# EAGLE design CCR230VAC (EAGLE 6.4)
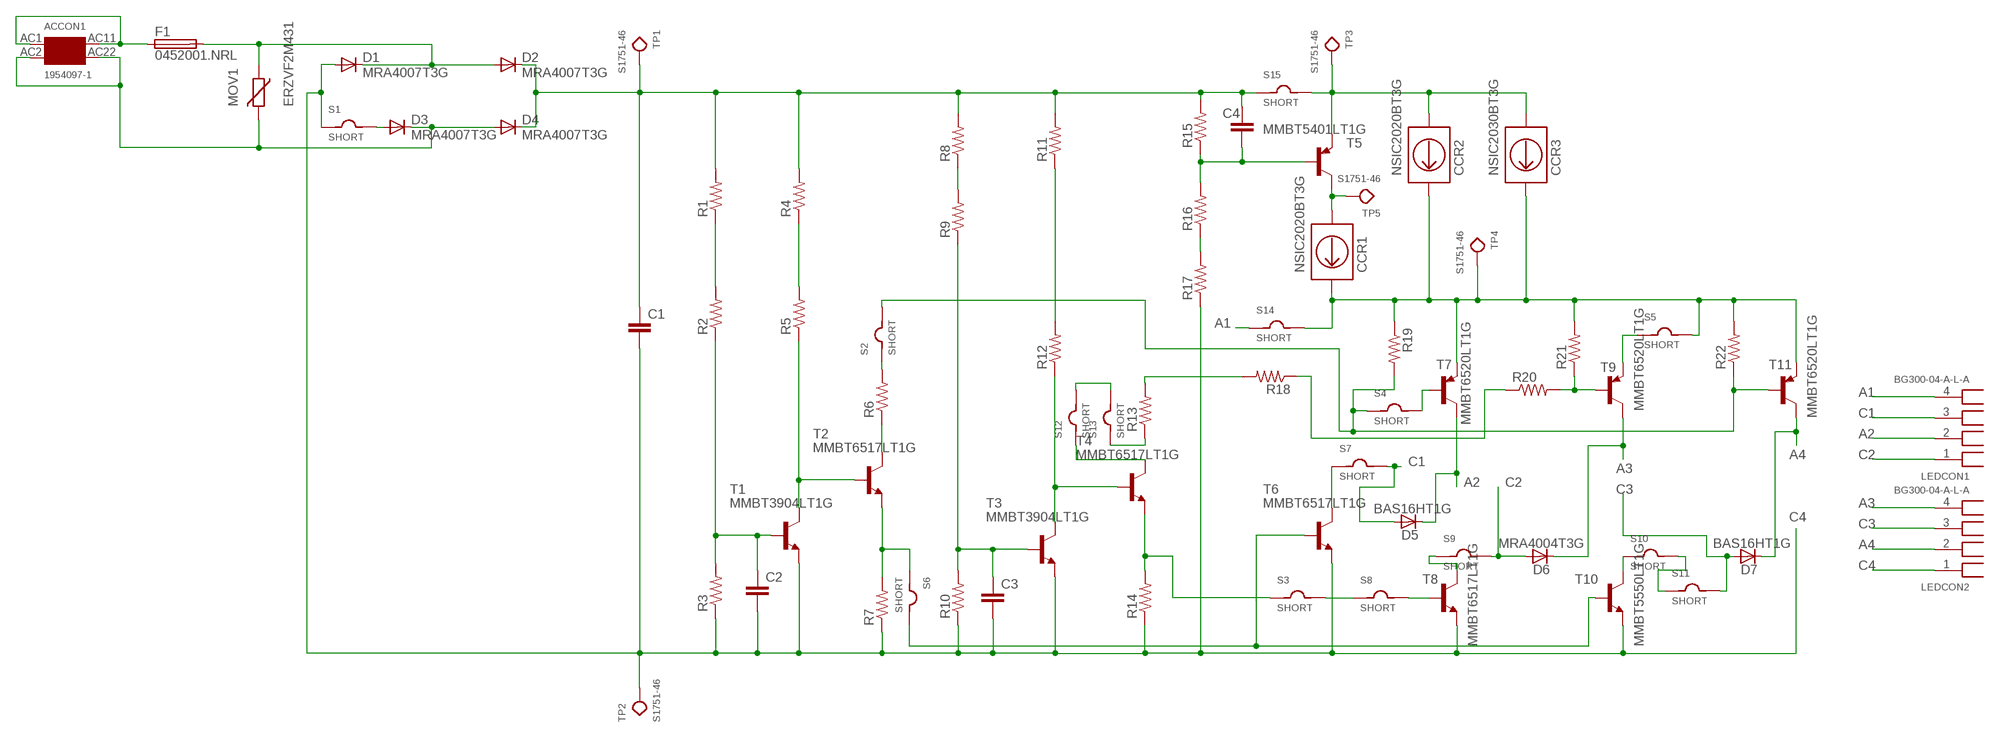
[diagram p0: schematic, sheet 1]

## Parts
ACCON1  1954097-1  [LEDCON_SMT]
C1  C-EUC1206K  [C1206K]
C2  C-EUC0805K  [C0805K]
C3  C-EUC0805K  [C0805K]
C4  C-EUC0805K  [C0805K]
CCR1  NSIC2020BT3G  NSIC2030BT3G  [SMB]
CCR2  NSIC2020BT3G  NSIC2030BT3G  [SMB]
CCR3  NSIC2030BT3G  [SMB]
D1  MRA4007T3G  MRA4004T3G  [SMA]
D2  MRA4007T3G  MRA4004T3G  [SMA]
D3  MRA4007T3G  MRA4004T3G  [SMA]
D4  MRA4007T3G  MRA4004T3G  [SMA]
D5  BAS16HT1G  [SOD323-R]
D6  MRA4004T3G  [SMA]
D7  BAS16HT1G  [SOD323-R]
F1  0452001.NRL  [SMTFUSE]
LEDCON1  BG300-04-A-L-A  [LEDCON_4_F]
LEDCON2  BG300-04-A-L-A  [LEDCON_4_F]
MOV1  ERZVF2M431  ERZVF2M241  [CU3225K]
R1  R-US_R1206  [R1206]
R2  R-US_R1206  [R1206]
R3  R-US_R1206  [R1206]
R4  R-US_R1206  [R1206]
R5  R-US_R1206  [R1206]
R6  R-US_R1206  [R1206]
R7  R-US_R1206  [R1206]
R8  R-US_R1206  [R1206]
R9  R-US_R1206  [R1206]
R10  R-US_R1206  [R1206]
R11  R-US_R1206  [R1206]
R12  R-US_R1206  [R1206]
R13  R-US_R1206  [R1206]
R14  R-US_R1206  [R1206]
R15  R-US_R1206  [R1206]
R16  R-US_R1206  [R1206]
R17  R-US_R1206  [R1206]
R18  R-US_R1206  [R1206]
R19  R-US_R1206  [R1206]
R20  R-US_R1206  [R1206]
R21  R-US_R1206  [R1206]
R22  R-US_R1206  [R1206]
S1  SHORT  [R2010]
S2  SHORT  [R2010]
S3  SHORT  [R2010]
S4  SHORT  [R2010]
S5  SHORT  [R2010]
S6  SHORT  [R2010]
S7  SHORT  [R2010]
S8  SHORT  [R2010]
S9  SHORT  [R2010]
S10  SHORT  [R2010]
S11  SHORT  [R2010]
S12  SHORT  [R2010]
S13  SHORT  [R2010]
S14  SHORT  [R2010]
S15  SHORT  [R2010]
T1  MMBT3904LT1G  [SOT23]
T2  MMBT6517LT1G  [SOT23]
T3  MMBT3904LT1G  [SOT23]
T4  MMBT6517LT1G  [SOT23]
T5  MMBT5401LT1G  [SOT23]
T6  MMBT6517LT1G  [SOT23]
T7  MMBT6520LT1G  [SOT23]
T8  MMBT6517LT1G  [SOT23]
T9  MMBT6520LT1G  [SOT23]
T10  MMBT5550LT1G  [SOT23]
T11  MMBT6520LT1G  [SOT23]
TP1  S1751-46  [TEST_SMT]
TP2  S1751-46  [TEST_SMT]
TP3  S1751-46  [TEST_SMT]
TP4  S1751-46  [TEST_SMT]
TP5  S1751-46  [TEST_SMT]

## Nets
A1: LEDCON1.4 S14.1
A2: D5.C LEDCON1.2 T7.3(C)
A3: D6.C LEDCON2.4 T9.3(C)
A4: D7.C LEDCON2.2 T11.3(C)
C1: D5.A LEDCON1.3 S7.2
C2: D6.A LEDCON1.1 S9.2
C3: D7.A LEDCON2.3 S11.2
C4: C1.2 C2.2 C3.2 D1.A LEDCON2.1 R3.1 R7.1 R10.1 R14.1 R17.1 S1.1 T1.2(E) T3.2(E) T6.2(E) T8.2(E) T10.2(E) TP2.P$1
CONECT: R19.2 R22.1 S2.2 S4.1 T11.1(B)
DDD: CCR1.C CCR2.C CCR3.C R19.1 R21.2 R22.2 S5.2 S14.2 T7.2(E) T11.2(E) TP4.P$1
N$1: ACCON1.AC1 ACCON1.AC11 F1.P$1
N$2: ACCON1.AC2 ACCON1.AC22 D3.C D4.A MOV1.2
N$3: D1.C D2.A F1.P$2 MOV1.1
N$4: D3.A S1.2
N$5: C4.2 R15.1 R16.2 T5.1(B)
N$6: R1.1 R2.2
N$7: C1.1 C4.1 D2.C D4.C R1.2 R4.2 R8.2 R11.2 R15.2 S15.1 TP1.P$1
N$8: R4.1 R5.2
N$9: C2.1 R2.1 R3.2 T1.1(B)
N$10: R5.1 T1.3(C) T2.1(B)
N$11: R16.1 R17.2
N$12: S6.2 T6.1(B) T10.1(B)
N$13: R6.2 S2.1
N$14: R6.1 T2.3(C)
N$15: R8.1 R9.2
N$16: C3.1 R9.1 R10.2 T3.1(B)
N$17: R20.2 R21.1 T9.1(B)
N$18: CCR1.A T5.3(C) TP5.P$1
N$19: R11.1 R12.2
N$20: R12.1 T3.3(C) T4.1(B)
N$21: R14.2 S3.1 T4.2(E)
N$22: S12.1 T4.3(C)
N$23: S3.2 S8.1
N$24: S5.1 T9.2(E)
N$25: R13.2 R18.2
N$26: R18.1 R20.1
N$27: S4.2 T7.1(B)
N$28: R7.2 S6.1 T2.2(E)
N$29: S7.1 T6.3(C)
N$30: S8.2 T8.1(B)
N$31: S9.1 T8.3(C)
N$32: S10.1 T10.3(C)
N$33: S10.2 S11.1
N$34: R13.1 S13.1
N$35: S12.2 S13.2
N$36: CCR2.A CCR3.A S15.2 T5.2(E) TP3.P$1

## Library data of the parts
ACCON1 = CCR_120VAC_LIB:1954097-1
C1-C4 = resistor:C-EU: CAPACITOR, European symbol
CCR1-CCR3 = CCR_120VAC_LIB:NSIC2030BT3G
D1-D4 D6 = CCR_120VAC_LIB:MRA4004T3G
D5 D7 = CCR_120VAC_LIB:BAS16HT1G
F1 = CCR_120VAC_LIB:0452001.NRL
LEDCON1 LEDCON2 = CCR_120VAC_LIB:BG300-04-A-L-A
MOV1 = CCR_120VAC_LIB:ERZVF2M241
R1-R22 = resistor:R-US_: RESISTOR, American symbol
S1-S15 = CCR_120VAC_LIB:SHORT
T1 T3 = CCR_120VAC_LIB:MMBT3904LT1G
T2 T4 T6 T8 = CCR_120VAC_LIB:MMBT6517LT1G
T5 = CCR_120VAC_LIB:MMBT5401LT1G
T7 T9 T11 = CCR_120VAC_LIB:MMBT6520LT1G
T10 = CCR_120VAC_LIB:MMBT5550LT1G
TP1-TP5 = CCR_120VAC_LIB:S1751-46

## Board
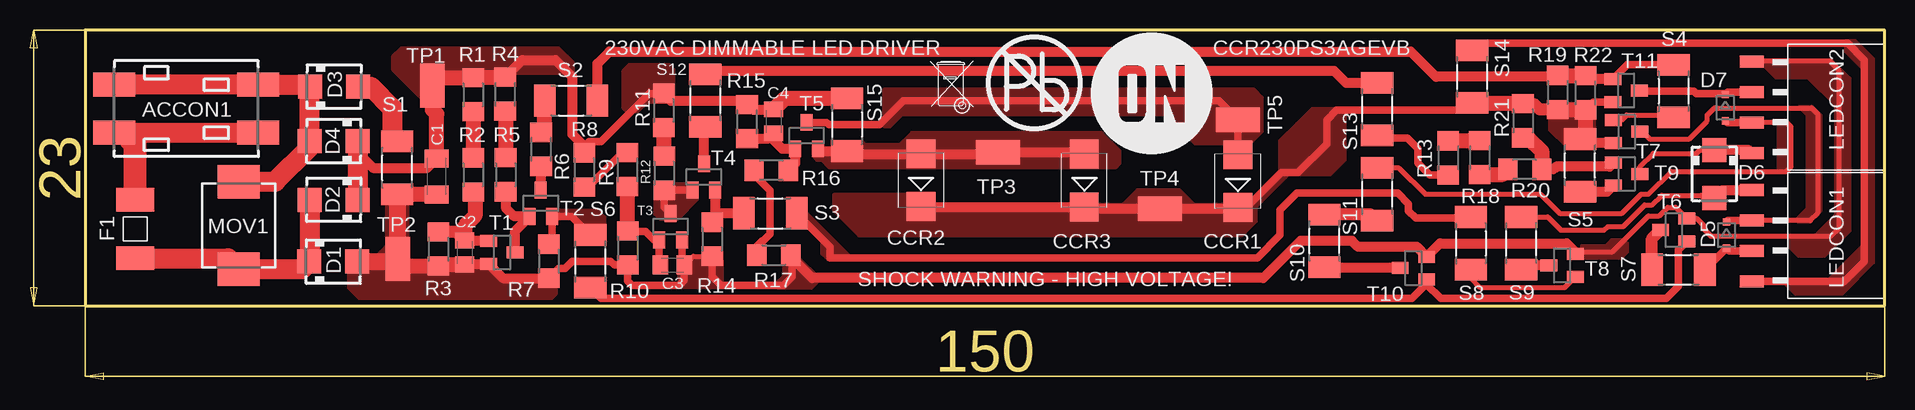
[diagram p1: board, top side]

Size 154.6 x 29.2 mm. Coordinates in mm from the lower left corner, seen from the top.
Outline: 4.6,6.2 154.6,6.2 154.6,29.2 4.6,29.2 4.6,6.2
Copper layers (1*16): Top 0.035mm / dielectric 1.5mm / Bottom 0.035mm
Design rules "default": minimum track width 10mil, minimum drill 24mil, track to track 8mil, track to pad 8mil, pad to pad 8mil, via to via 8mil, smd to smd 8mil, copper to edge 1mil, drill to drill 8mil, minimum pad ring 10mil, minimum via ring 8mil, stop-mask expansion 4mil, vias tented up to drill 0mil, thermal gap 10mil

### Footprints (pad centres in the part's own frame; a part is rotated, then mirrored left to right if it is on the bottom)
LEDCON_SMT = smd 3.5 x 2: AC1 -6,2; AC2 -6,-2; AC11 6,2; AC22 6,-2
C1206K = smd 1.5 x 2: 1 -1.5,0; 2 1.5,0
C0805K = smd 1.3 x 1.6: 1 -1,0; 2 1,0
SMB = smd 2.4 x 2.4: A 2.2,0; C -2.2,0
SMA = smd 2 x 2: A 2,0; C -2,0
SOD323-R = smd 0.6 x 0.6: A 1.1,0; C -1.1,0
SMTFUSE = smd 1.96 x 3.15: P$1 -2.45,0; P$2 2.45,0
LEDCON_4_F = smd 2 x 1: 1 0,2.54; 2 0,0; 3 0,-2.54; 4 0,-5.08
CU3225K = smd 2.8 x 3.5: 1 -3.65,0; 2 3.65,0
R1206 = smd 1.6 x 1.803: 1 -1.422,0; 2 1.422,0
R2010 = smd 1.8 x 2.7: 1 -2.2,0; 2 2.2,0
SOT23 = smd 1 x 1.4: 1 -0.95,-1.1; 2 0.95,-1.1; 3 0,1.1
TEST_SMT = smd 3.65 x 2.05: P$1 0,0

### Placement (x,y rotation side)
ACCON1  13.03,22.62 180 top
C1  33.91,16.99 270 top
C2  36.24,10.64 270 top
C3  53.55,9.59 0 top
C4  61.99,21.56 270 top
CCR1  100.68,16.58 90 top
CCR2  74.28,16.66 90 top
CCR3  87.88,16.64 90 top
D1  25.29,9.87 0 top
D2  25.33,15.03 180 top
D3  25.35,24.47 0 top
D4  25.32,19.93 180 top
D5  141.41,12.09 270 top
D6  140.4,17.2 270 top
D7  141.31,22.71 270 top
F1  8.77,12.59 270 top
LEDCON1  143.5,13.3 0 top
LEDCON2  143.5,24 0 top
MOV1  17.39,12.9 90 top
R1  36.95,23.81 90 top
R2  36.95,17.11 90 top
R3  34.05,10.93 90 top
R4  39.6,23.85 90 top
R5  39.65,17.12 90 top
R6  42.6,19.24 90 top
R7  43.25,9.91 90 top
R8  46.2,17.53 90 top
R9  49.8,17.55 90 top
R10  49.82,11.01 90 top
R11  52.82,22.48 90 top
R12  52.87,17.25 90 top
R13  118.22,18.52 90 top
R14  56.87,11.74 90 top
R15  59.77,21.56 90 top
R16  61.78,17.48 0 top
R17  62,10.42 180 top
R18  120.84,18.56 90 top
R19  127.34,23.98 90 top
R20  124.6,17.56 0 top
R21  124.44,21.62 90 top
R22  129.66,23.96 270 top
S1  30.6,17.7 90 top
S2  45.1,23.3 0 top
S3  61.7,13.9 0 top
S4  137,24.1 270 top
S5  129.2,17.9 90 top
S6  46.7,9.9 270 top
S7  137.4,9.2 0 top
S8  120.1,11.4 270 top
S9  124.3,11.4 90 top
S10  107.9,11.6 90 top
S11  112.3,15.5 90 top
S12  56.3,23.3 90 top
S13  112.3,22.6 90 top
S14  120.2,25.3 270 top
S15  68.1,21.3 270 top
T1  39.34,10.64 270 top
T2  42.58,14.74 0 top
T3  53.4,12.79 0 top
T4  56.17,16.94 0 top
T5  64.74,20.39 0 top
T6  137.01,12.51 90 top
T7  133.09,20.72 270 top
T8  127.71,9.55 90 top
T9  133.09,17.19 270 top
T10  115.31,9.33 90 top
T11  133.04,24.15 270 top
TP1  33.55,24.55 270 top
TP2  30.65,10.1 270 top
TP3  80.7,19 0 top
TP4  94.2,14.3 0 top
TP5  100.7,21.7 0 top
U$1  [ON2]  93.5,23.9 0 top
U$2  [BIN2]  76.8,24.5 0 top
U$3  [PB1]  83.7,24.8 0 top

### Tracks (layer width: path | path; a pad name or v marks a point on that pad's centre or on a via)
A1
  Top 0.61: S14.1 120.8,28.1 151.5,28.1 152.9,26.7 152.9,9.9 151.22,8.22 LEDCON1.4
  pour Top: 146.2,8.2 146.2,8.1 147.1,7.2 151.1,7.2 153.7,9.8 153.7,26.8 152.3,28.2 152.2,28.3 151.3,28.3 151.3,27.4 152.7,26 152.7,11.2 149.9,8.4 146.2,8.4
A2
  Top 0.406: LEDCON1.2 148.4,13.3 149,13.9 149,22.2 148.5,22.7 140.4,22.7 139.8,22.1 139.8,21.6 138.3,20.1 135,20.1 134.38,20.72 T7.3
  Top 0.61: LEDCON1.2 141.52,13.3 D5.C
  pour Top: 147.3,13.2 148.4,13.2 149.3,14.1 149.3,22.1 148.6,22.8 147.4,22.8 148.1,22.1 148.1,14.3 147.3,13.5
A3
  Top 0.406: T9.3 134.19,17.79 135.3,18.9 138.9,18.9 139.2,19.2 D6.C
  Top 0.813: LEDCON2.4 143.22,19.2 D6.C
A4
  Top 0.61: LEDCON2.2 141.5,24 D7.C 141.22,23.9 138.9,23.9 138.7,24.1 134.19,24.1 T11.3
C1
  Top 0.61: S7.2 139.62,9.2 D5.A 141.64,10.76 LEDCON1.3
C2
  Top 0.406: S9.2 126.5,13.6 127.6,12.5 131.2,12.5 131.5,12.8 132.8,12.8 134.6,14.6 135.2,14.6 136,15.4 139.3,15.4 139.5,15.2 D6.A
  Top 0.813: D6.A 141.04,15.84 LEDCON1.1
C3
  Top 0.406: S11.2 114.1,17.7 116.3,15.5 125.9,15.5 127.5,13.9 132.7,13.9 134.3,15.5 134.9,15.5 136.8,17.4 146.4,17.4 146.8,17.8 146.8,21.1 146.44,21.46 LEDCON2.3
  Top 0.61: D7.A 141.46,21.46 LEDCON2.3
  pour Top: 145.7,21.4 145.7,17.4 146.4,17.4 146.8,17.8 146.8,21.1 146.4,21.5 145.8,21.5
C4
  Top 0.406: C3.2 55.28,10.32 R14.1 | 128.81,10.69 131.89,10.69 134.9,13.7 135.8,13.7 136.5,14.4 137.17,14.4 T6.2 138.94,13.46 139.5,12.9 139.5,12.6 140.1,12 150.1,12 150.8,12.7 150.8,25.8 150,26.6 143.56,26.6 LEDCON2.1
  Top 0.61: R7.1 44.06,9.3 44.6,9.3 45.2,9.9 48.4,9.9 48.71,9.59 R10.1 49.82,8.28 50.2,7.9 54.1,7.9 54.5,8.3 54.5,9.54 C3.2 54.35,9.79 T3.2 | R14.1 56.87,8.63 57.6,7.9 62.8,7.9 63.5,8.6 63.5,10.34 R17.1
  Top 0.813: C2.2 38.19,9.64 T1.2 39.44,8.49 R7.1 | T8.2 128.81,10.69 128.1,11.4 117.53,11.4 T10.2 115.59,11.1 110.7,11.1 110.2,11.6 105.9,11.6 102.8,8.5 65.2,8.5 63.42,10.28 R17.1
  Top 1.27: S1.1 C1.2 | TP2.P$1 31.24,9.51 R3.1 34.18,9.64 C2.2
  Top 1.422: S1.1 30.6,10.15 TP2.P$1 30.42,9.87 D1.A
  pour Top (no thermals): 26.5,10 26.5,7.7 27.4,6.8 43.5,6.8 43.9,7.2 43.9,8.3 43.5,8.7 39.3,8.7 38.2,9.8 31.8,9.8 31.5,10.1 31.5,15 31.3,15.2 29.9,15.2 29.7,15 29.7,11.2 28.9,10.4 26.9,10.4
  pour Top (no thermals): 54.1,10.2 57.5,10.2 57.7,10 57.7,7.9 57.5,7.7 54.3,7.7 54.1,7.9
  pour Top (no thermals): 129.3,10.2 132.7,10.2 133.2,10.7 133.2,11.4 132.9,11.7 131.8,11.7 131.3,11.2 129.3,11.2
  pour Top (no thermals): 144.3,26.7 150.2,26.7 151.7,25.2 151.7,12.4 149.6,10.3 147.4,10.3 146.7,11 146.7,11.7 147.1,12.1 148.8,12.1 150.5,13.8 150.5,22.9 148.2,25.2 145.5,25.2 144.5,26.2 144.3,26.2
  pour Top (no thermals): 62.8,9.8 62.8,8.7 62.2,8.1 62.2,7.8 62.3,7.7 65.2,7.7 65.8,8.3 65.8,8.5 64.1,10.2 64.1,11.2 62.8,11.2
CONECT
  Top 0.61: T11.1 133.14,26.3 S4.1
  Top 0.813: S2.2 47.3,26.4 48.3,27.4 115.1,27.4 117.2,25.3 127.24,25.3 R19.2 | T11.1 129.94,25.1 R22.1
  Top 1.27: R19.2 129.64,25.4 R22.1
DDD
  Top 0.61: T11.2 130.32,23.2 R22.2 | CCR1.C 101.38,14.38 104.3,17.3 105.7,17.3 108.1,19.7 108.1,21.7 108.9,22.5 119.6,22.5 S14.2
  Top 0.813: T7.2 129.53,19.77 S5.2 | CCR2.C 74.3,14.44 CCR3.C 88.02,14.3 TP4.P$1 100.6,14.3 CCR1.C
  Top 1.016: R19.1 125.84,22.56 125.4,23 124.48,23 R21.2
  Top 1.27: R19.1 129.64,22.56 R22.2 129.66,20.56 S5.2 | R21.2 120.26,23.04 S14.2
  pour Top (no thermals): 126.7,23.1 130.2,23.1 130.4,22.9 130.4,19.7 130.2,19.5 128,19.5 126.7,20.8
  pour Top (no thermals): 67,15.5 74.5,15.5 75.3,14.7 91.1,14.7 92.3,15.9 95.8,15.9 97,14.7 101.4,14.7 104.2,17.5 104.2,20 105.6,21.4 106.9,22.7 108.6,22.7 109,22.7 109.6,22.1 109.6,18.3 108.4,17.1 104.9,17.1 102.2,14.4 102.2,13.2 101,12 69.1,12 67,14.1
N$1
  Top 1.676: ACCON1.AC11 7.85,20.62 ACCON1.AC1
  Top 1.93: F1.P$1 8.77,19.7 7.85,20.62
N$2
  Top 1.676: ACCON1.AC22 ACCON1.AC2 23.2,24.62 D3.C 23.32,24.44 D4.A 23.3,19.91 23.3,19.4 20.45,16.55 MOV1.2
N$3
  Top 1.676: F1.P$2 16.5,10.14 MOV1.1 22.67,9.25 D1.C 23.33,9.91 D2.A
N$4
  Top 1.676: D3.A 28.43,24.47 30.2,22.7 30.2,20.3 S1.2
N$5
  Top 0.813: R15.1 61.57,20.14 C4.2 61.99,20.01 62.7,19.3 T5.1 63.79,18.07 R16.2
N$6
  Top 1.27: R1.1 R2.2
N$7
  Top 0.61: R11.2 51.6,23.9 47.6,19.9 46.6,19.9 46.2,19.5
  Top 0.813: D4.C 27.32,18.98 28.6,17.7 33.12,17.7 C1.1 | R4.2 41.03,26.7 43.8,26.7 45.2,25.3 45.2,20.5 46.2,19.5 R8.2 | R11.2 53.42,23.3 59.2,23.3 59.52,22.98 R15.2 60.19,22.56 C4.1
  Top 1.27: C1.1 33.9,22.2 33.55,22.55 TP1.P$1 34.23,25.23 R1.2 36.99,25.27 R4.2 | C4.1 62.93,23.5 S15.1
  Top 1.676: D4.C D2.C
  pour Top (no thermals): 53.7,23.8 53.7,25.9 53.3,26.3 49.9,26.3 49.4,25.8 49.4,22.7 49.7,22.4 50.7,22.4 51.4,23.1 51.5,23.2 53.1,23.2
  pour Top (no thermals): 45.3,25.6 45.3,26.5 44.1,27.7 30.9,27.7 30.2,27 30.2,25.9 33.2,22.9 33.9,22.9 34.4,23.4 34.4,24.6 34.6,24.8 39.5,24.8 40.3,25.6
N$8
  Top 1.27: R4.1 39.65,22.38 R5.2
N$9
  Top 0.813: T1.1 36.29,11.59 C2.1
  Top 1.016: C2.1 35.53,12.35 R3.2
  Top 1.27: R2.1 37.1,15.54 37.1,13.7 36.24,12.84 C2.1
N$10
  Top 0.813: T1.3 40.44,12.45 T2.1 40.36,13.64 39.7,14.3 39.7,15.65 R5.1
N$11
  Top 0.61: R16.1 60.36,17.14 61.7,15.8 61.7,12.2 61.1,11.6 61,11.6 60.6,11.2 60.6,10.44 R17.2
N$12
  Top 0.61: T6.1 137.4,10.85 137.4,7.8 136.4,6.8 117.6,6.8 116.41,7.99 T10.1 116.41,8.01 115.2,6.8 47.6,6.8 S6.2
N$13
  Top 1.27: R6.2 42.9,20.96 S2.1
N$14
  Top 0.813: T2.3 42.6,15.86 R6.1
N$15
  Top 0.61: R8.1 46.51,16.11 49,18.6 49.43,18.6 R9.2
N$16
  Top 0.61: C3.1 52.45,9.69 T3.1 52.01,11.69 51.3,12.4 49.85,12.4 R10.2 | 49.82,16.11 R9.1
  Top 1.27: R10.2 49.82,16.11
N$17
  Top 0.813: T9.1 131.65,17.8 127.2,17.8 126.96,17.56 R20.2
  Top 1.27: R21.1 124.9,20.2 126,19.1 126,17.58 R20.2
N$18
  Top 0.61: T5.3 66.41,21.49 66.6,21.3 70.8,21.3 72.8,23.3 99.1,23.3 TP5.P$1 100.68,21.68 CCR1.A
  pour Top (no thermals): 71.2,24.3 102,24.3 102.7,23.6 102.7,20.7 101.7,19.7 97.1,19.7 94.7,22.1 72.7,22.1 71.7,21.1 71.2,21.1
N$19
  Top 0.61: 52.82,18.72 R12.2
  Top 1.27: R11.1 52.82,18.72
N$20
  Top 0.61: T3.3 52.87,14.42 R12.1 55.21,15.83 T4.1
  pour Top (no thermals): 52.2,16.4 55.4,16.4 55.6,16.2 55.6,15 54,13.4 52.5,13.4 52.1,13.8 52.1,16.3
N$21
  Top 0.813: T4.2 57.12,13.41 R14.2 57.61,13.9 S3.1
N$22
  Top 0.813: T4.3 56.17,20.97 S12.1
N$23
  Top 0.61: S8.1 120,13.5 115.5,13.5 114.9,14.1 114.9,14.7 114,15.6 105.6,15.6 104.2,14.2 104.2,12.1 102.3,10.2 66.7,10.2 66.7,11.1 S3.2
  pour Top (no thermals): 64.6,15.1 64.6,14.1 68.3,10.4 68.3,10.2 68.1,10 66.5,10 66,10.5 66,11.5 64.6,12.9 63.2,12.9 63.2,14.8 63.5,15.1
N$24
  Top 0.813: T9.2 131.45,15.7 S5.1
N$25
  Top 1.27: R13.2 118.26,19.98 R18.2
N$26
  Top 1.27: R18.1 122.76,17.14 R20.1
N$27
  Top 0.406: T7.1 132.02,21.7 132.7,21.7 133.1,22.1 136.8,22.1 S4.2
N$28
  Top 0.61: R7.2 43.53,11.61 T2.2 45.16,13.64 S6.1
  pour Top (no thermals): 43.3,14.2 47.3,14.2 47.9,13.6 47.9,11.8 47.6,11.5 46.2,11.5 45.7,12 45.7,12.9 45.1,13.5 43.3,13.5
N$29
  Top 1.016: S7.1 135.2,11.8 T6.3
N$30
  Top 0.406: T8.1 127.91,7.7 120.9,7.7 120.1,8.5 S8.2
N$31
  Top 0.813: T8.3 124.65,9.55 S9.1
N$32
  Top 0.813: S10.1 114.14,9.4 T10.3
N$33
  Top 1.016: S11.1 111.8,13.8 S10.2
N$34
  Top 0.61: R13.1 116.7,17.1 115.7,18.1 115.7,19.3 114.8,20.2 112.5,20.2 S13.1
N$35
  Top 0.813: S12.2 56.6,25.8 108.7,25.8 109.7,24.8 S13.2
N$36
  Top 0.813: T5.2 65.88,19.1 S15.2 68.34,18.86 CCR2.A 80.56,18.86 TP3.P$1 87.72,19 CCR3.A
  pour Top (no thermals): 69.4,19.9 69.6,19.7 72.5,19.7 73.5,20.7 89.3,20.7 90.8,19.2 90.8,18 90.5,17.7 66.6,17.7 66,18.3 65.6,18.3 65.3,18.6 65.3,19 65.6,19.3 67,19.3 67.5,19.8 67.5,19.9

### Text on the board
tNames: 230VAC DIMMABLE LED DRIVER | CCR230PS3AGEVB | SHOCK WARNING - HIGH VOLTAGE!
